// TwinCAT 3 PLC project TcComProxy
// ProgramVersion: 3.1.4024.0
// libraries:
//   Tc2_Standard, * (Beckhoff Automation GmbH)
//   Tc2_System, * (Beckhoff Automation GmbH)
//   Tc2_Utilities, * (Beckhoff Automation GmbH)
//   Tc3_Module, * (Beckhoff Automation GmbH)
//   TcComProxyApplication, * (YuYang_Beckhoffsh)
// project tree:
//   / PlcTask.TcTTO
//   POUs/ FB_ProxyTcComIncrementModule.TcPOU, MAIN.TcPOU
// (motion and I/O tree: see PLC project dyntccomproxy)
// real-time tasks:
//   TASK PlcTask: cycle T#10ms, priority 20, ADS port 350
//   TASK PlcTask1: cycle T#10ms, priority 21, ADS port 351
//   TASK PlcTask2: cycle T#10ms, priority 22, ADS port 352
//   TASK PlcTask3: cycle T#10ms, priority 23, ADS port 353
// variable links:

CONFIGURATION TcComProxy
    RESOURCE PLC ON TwinCAT3
        TASK PlcTask(INTERVAL := T#10ms, PRIORITY := 21);
        PROGRAM MAIN WITH PlcTask : MAIN;
    END_RESOURCE
END_CONFIGURATION

// ---- POUs/MAIN.TcPOU
PROGRAM MAIN
VAR
	fbProxyTcComIncrementModule	: FB_ProxyTcComIncrementModule(	IID	:= TC_GLOBAL_IID_LIST.IID_IIncrement);
	nValue: INT;
END_VAR

IF fbProxyTcComIncrementModule.ip <> 0 THEN
	
	fbProxyTcComIncrementModule.Cyclic();
	fbProxyTcComIncrementModule.ip.doIncrement(1,ADR(nValue));
	
END_IF

END_PROGRAM

// ---- POUs/FB_ProxyTcComIncrementModule.TcPOU
FUNCTION_BLOCK FB_ProxyTcComIncrementModule EXTENDS FB_ProxyTcComModule
VAR_INPUT
END_VAR
VAR_OUTPUT
END_VAR
VAR
	_iThisProvider		: IIncrement;
END_VAR

METHOD FB_exit : BOOL
VAR_INPUT
	bInCopyCode : BOOL; // if TRUE, the exit method is called for exiting an instance that is copied afterwards (online change).
END_VAR
IF NOT bInCopyCode THEN
	FW_SafeRelease(pipUnk:= ADR(_iThisProvider));
END_IF
END_METHOD

METHOD FB_init : BOOL
VAR_INPUT
	bInitRetains 	: BOOL; // if TRUE, the retain variables are initialized (warm start / cold start)
	bInCopyCode 	: BOOL;  // if TRUE, the instance afterwards gets moved into the copy code (online change)
	IID				: IID;
END_VAR
ComQueryInterface(Super^._iProvider,TC_GLOBAL_IID_LIST.IID_IIncrement, ADR(_iThisProvider));
END_METHOD

PROPERTY ip : IIncrement
GET
ip	:= _iThisProvider;
END_GET
END_PROPERTY

END_FUNCTION_BLOCK
